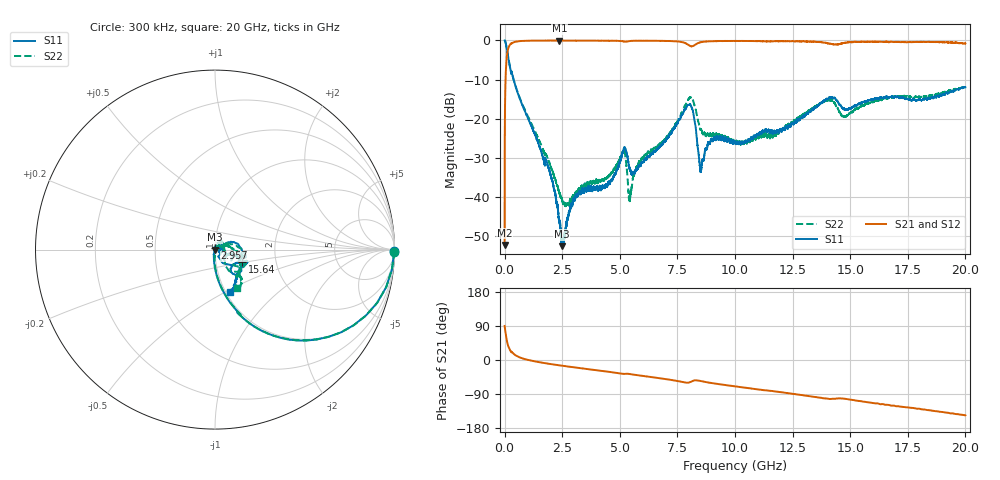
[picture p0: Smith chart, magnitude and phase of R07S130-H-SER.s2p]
!{R07S130}
!Johanson Technology Inc.
!www.johansontechnology.com
!Test Board Conditions:
!Substrate Type  RO4350B
!Substrate Thickness  10 mil
!Substrate Dk  3.66
!TL Type: GCPW
!TL Trace Width  21 mil
!TL Gap  20 mil
!Electrode orientation  Horizontal
!DUT TOPOLOGY	SERIES
!Mounting Pad LxW  16x21 mil
! Created Sat Feb  6 11:45:57 2021
# hz S ma R 50
! 2 Port Network Data from SP1.SP block
! freq  magS11  angS11  magS21  angS21  magS12  angS12  magS22  angS22
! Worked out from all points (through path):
!   20001 points, 300 kHz to 20 GHz, reference 50 ohm
!   highest |S21| = -0.02 dB at 2.381 GHz (marker M1); lowest = -52.1 dB at 300 kHz (marker M2)
!   group delay of S21, straight-line fit = 21.2 ps
!   lowest |S11| = -52.5 dB at 2.477 GHz (marker M3), VSWR 1.00, Z = 49.8 - j0.103 ohm
!   |S11| at or under -10 dB: 390.8 MHz to end of sweep
!   |S22| runs from -42.3 to 0.0 dB; largest |S21 - S12| = 0.013
!   S11 on the Smith chart (normalised r, x): 300 kHz: open; 2.957 GHz: 1.00, +0.02; 15.64 GHz: 1.34, -0.19; 20 GHz: 1.05, -0.53
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300000  0.9981 -0.5  0.00247 89.9  0.002431 88.9  1 -0.7
1.043e8  0.7569 -41.4  0.6483 49.0  0.65 48.9  0.7585 -41.2
2.123e8  0.4945 -62.0  0.8657 28.5  0.8647 28.5  0.4945 -62.0
6.073e8  0.1998 -81.8  0.9772 8.1  0.9771 8.2  0.2023 -81.3
1.8873e9  0.02436 -101.3  0.9971 -9.7  0.9961 -9.7  0.02984 -93.4
2.3813e9  0.004989 -129.7  0.9974 -14.0  0.9956 -14.1  0.01135 -71.7
2.4773e9  0.002377 -154.3  0.9964 -14.9  0.9962 -14.9  0.00974 -59.5
2.9573e9  0.008435 98.7  0.9962 -18.9  0.9954 -18.8  0.01028 -0.5
3.3343e9  0.01193 95.4  0.9949 -21.9  0.9956 -21.8  0.0139 11.3
4.5023e9  0.01542 63.9  0.9916 -31.0  0.9917 -31.0  0.0181 43.6
5.1433e9  0.03864 13.7  0.9758 -36.5  0.9759 -36.5  0.038 34.5
5.4533e9  0.02206 -26.8  0.9846 -37.2  0.9855 -37.1  0.01048 56.2
5.7823e9  0.02343 -2.0  0.9905 -40.1  0.9909 -40.1  0.02547 79.7
6.6673e9  0.04201 18.0  0.9889 -47.5  0.9896 -47.6  0.04505 58.1
8.0663e9  0.1519 -21.3  0.848 -58.3  0.8472 -58.3  0.1885 -27.9
8.5343e9  0.0232 13.7  0.9518 -55.8  0.9523 -55.9  0.07277 -46.1
9.0333e9  0.05214 57.0  0.9803 -61.3  0.9778 -61.4  0.06338 -24.5
1.00003e10  0.05054 28.1  0.9851 -69.6  0.9856 -69.6  0.04894 0.6
1.33343e10  0.1291 -18.3  0.9644 -96.3  0.9657 -96.4  0.1354 -6.1
1.56383e10  0.1657 -23.9  0.9612 -110.4  0.9598 -110.4  0.1527 -24.7
1.66673e10  0.1858 -21.0  0.9515 -118.6  0.9573 -118.9  0.1871 -42.2
2e10  0.2533 -70.2  0.9137 -145.8  0.9066 -145.7  0.2502 -60.2
